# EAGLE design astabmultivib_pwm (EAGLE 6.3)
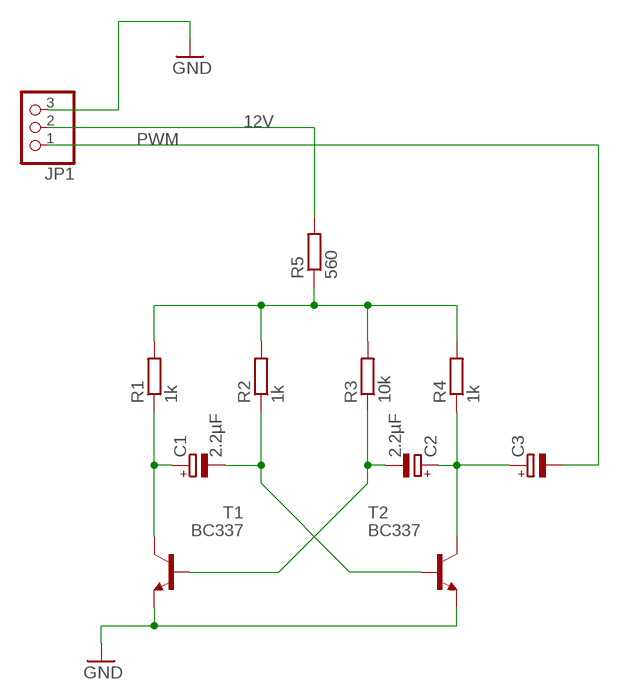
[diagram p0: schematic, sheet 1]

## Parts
C1  2.2µF  CPOL-EUE2.5-6  [E2,5-6]
C2  2.2µF  CPOL-EUE2.5-6  [E2,5-6]
C3  CPOL-EUE2.5-6  [E2,5-6]
JP1  PINHD-1X3/90  [1X03/90]
R1  1k  R-EU_0207/10  [0207/10]
R2  1k  R-EU_0207/10  [0207/10]
R3  10k  R-EU_0207/10  [0207/10]
R4  1k  R-EU_0207/10  [0207/10]
R5  560  R-EU_0207/10  [0207/10]
T1  BC337  [TO92]
T2  BC337  [TO92]

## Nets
12V: JP1.2 R5.2
GND: JP1.3 T1.1(E) T2.1(E)
N$1: R1.2 R2.2 R3.2 R4.2 R5.1
N$2: C2.- R3.1 T1.2(B)
N$3: C1.- R2.1 T2.2(B)
N$4: C1.+ R1.1 T1.3(C)
N$5: C2.+ C3.+ R4.1 T2.3(C)
PWM: C3.- JP1.1

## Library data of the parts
C1-C3 = rcl:CPOL-EU: POLARIZED CAPACITOR, European symbol
JP1 = pinhead:PINHD-1X3: PIN HEADER
R1-R5 = resistor:R-EU_: RESISTOR, European symbol
T1 T2 = transistor:BC337: NPN TRANSISTOR

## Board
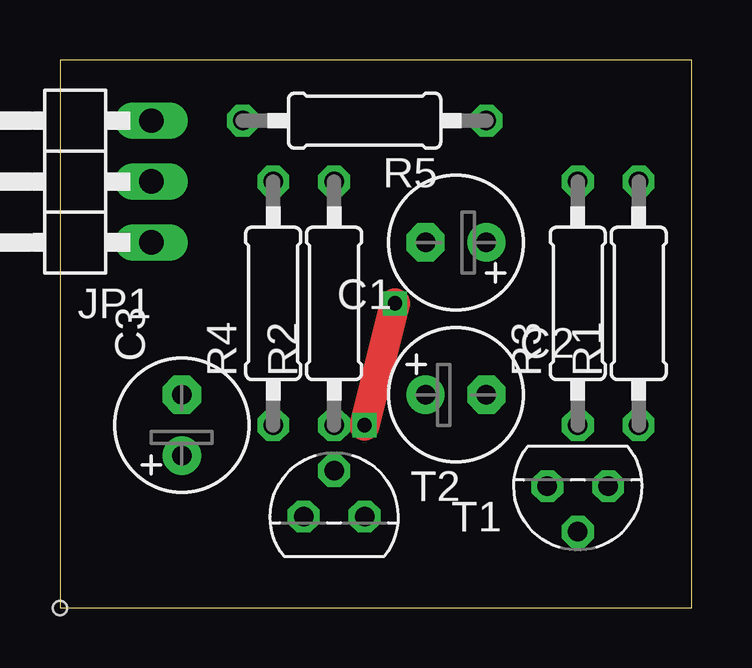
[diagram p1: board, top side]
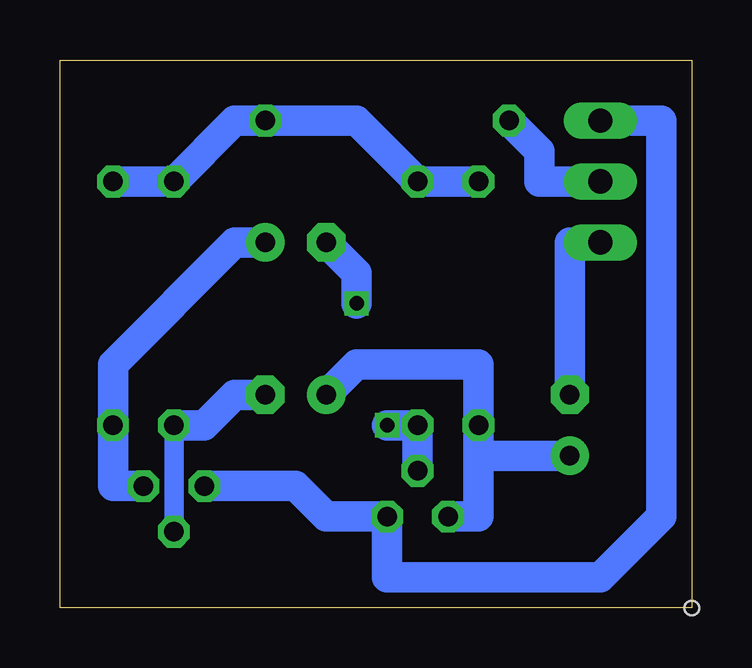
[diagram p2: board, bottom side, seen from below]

Size 26.34 x 22.85 mm. Coordinates in mm from the lower left corner, seen from the top.
Outline: 0,0 26.34,0 26.34,22.85 0,22.85 0,0
Copper layers (1*16): Top 0.035mm / dielectric 1.5mm / Bottom 0.035mm
Design rules "default": minimum track width 10mil, minimum drill 24mil, track to track 8mil, track to pad 8mil, pad to pad 8mil, via to via 8mil, smd to smd 8mil, copper to edge 40mil, drill to drill 8mil, minimum pad ring 10mil, minimum via ring 8mil, stop-mask expansion 4mil, vias tented up to drill 0mil, thermal gap 10mil
Holes 0.6 mm at 0,0

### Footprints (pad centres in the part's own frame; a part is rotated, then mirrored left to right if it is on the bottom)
E2,5-6 = drill 0.813 pad 1.6: + -1.27,0 | drill 0.813 pad 1.6 octagon: - 1.27,0
1X03/90 = drill 1.016 long: 1 -2.54,-3.81; 2 0,-3.81; 3 2.54,-3.81
0207/10 = drill 0.813 octagon: 1 -5.08,0; 2 5.08,0
TO92 = drill 0.813 octagon: 1 1.27,0; 2 0,1.905; 3 -1.27,0

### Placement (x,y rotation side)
C1  16.51,15.24 180 top
C2  16.51,8.89 0 top
C3  5.08,7.62 90 top
JP1  0,17.78 90 top
R1  24.13,12.7 90 top
R2  11.43,12.7 90 top
R3  21.59,12.7 90 top
R4  8.89,12.7 90 top
R5  12.7,20.32 180 top
T1  21.59,5.08 180 top
T2  11.43,3.81 0 top

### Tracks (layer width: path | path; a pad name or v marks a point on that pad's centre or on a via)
12V
  Bottom 1.27: JP1.2 6.35,17.78 6.35,19.05 R5.2
GND
  Bottom 1.27: T1.1 16.51,5.08 15.24,3.81 T2.1 12.7,1.27 3.81,1.27 1.27,3.81 1.27,20.32 JP1.3
N$1
  Bottom 1.27: R4.2 R2.2 13.97,20.32 R5.1 19.05,20.32 R3.2 R1.2
N$2
  Bottom 0.813: R3.1 T1.2
  Bottom 1.27: C2.- 19.05,8.89 20.32,7.62 R3.1
N$3  (via drill 0.6)
  Top 1.27: v13.97,12.7 v12.7,7.62
  Bottom 1.27: T2.2 R2.1 v12.7,7.62 | C1.- 13.97,13.97 v13.97,12.7
N$4
  Bottom 1.27: C1.+ 19.05,15.24 24.13,10.16 R1.1 24.13,5.08 T1.3
N$5
  Bottom 1.27: T2.3 8.89,3.81 8.89,6.35 | 8.89,6.35 R4.1 8.89,10.16 13.97,10.16 C2.+ | C3.+ 8.89,6.35
PWM
  Bottom 1.27: C3.- 5.08,15.24 JP1.1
